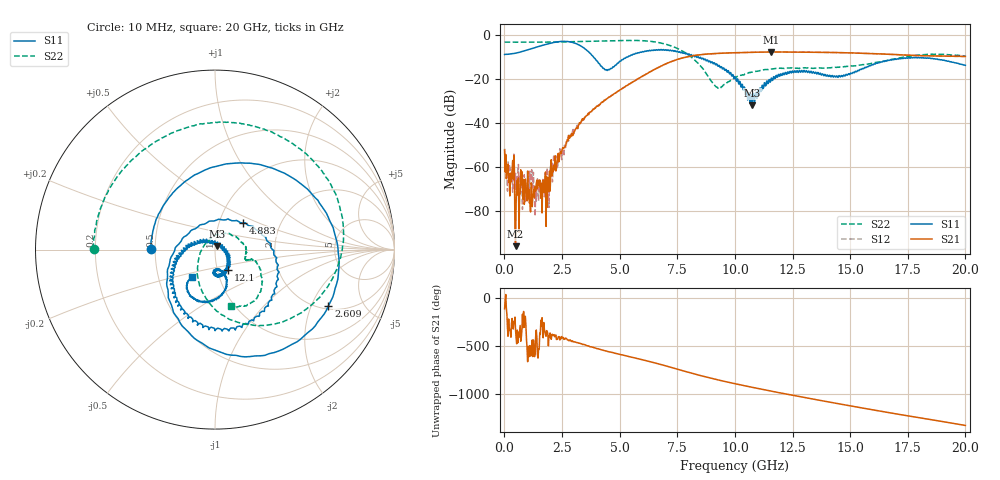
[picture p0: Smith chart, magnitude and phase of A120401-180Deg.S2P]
!  2-Port S-parameters saved by WinCal
! VAR MeasName=S-Parameters (CALIBRATED_DATA) read from VNA (N5244A)
! VAR MeasDate=11/21/2012 9:58:23 AM
! VAR NAME=A120401-180Deg
! VAR FILENAME=A120401-180Deg.S2P
! VAR DATE=11/21/2012 9:58:23 AM
! VAR PHYS_PORTS=1,2
# Hz S MA R 50
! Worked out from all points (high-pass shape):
!   801 points, 10 MHz to 20 GHz, reference 50 ohm
!   highest |S21| = -7.83 dB at 11.55 GHz (marker M1); lowest = -96.2 dB at 484.8 MHz (marker M2)
!   |S21| within 3 dB of the highest: 7.632 GHz to end of sweep
!   lowest |S11| = -32.1 dB at 10.75 GHz (marker M3), VSWR 1.05, Z = 51.3 + j2.13 ohm
!   |S11| at or under -10 dB: 3.858 GHz to 5.368 GHz (1.51 GHz wide, 32.7 % of centre); 8.329 GHz to 8.405 GHz (76.47 MHz wide, 0.914 % of centre); 8.406 GHz to end of sweep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
!   |S22| runs from -24.5 to -2.6 dB; largest |S21 - S12| = 0.0043
!   S11 on the Smith chart (normalised r, x): 10 MHz: 0.48, +0.00; 2.609 GHz: 2.14, -2.68; 4.883 GHz: 1.30, +0.41; 12.1 GHz: 1.13, -0.26; 20 GHz: 0.74, -0.24
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1e7  0.3546 179.4  0.002379 -112.7  0.002555 -35.3  0.6748 179.6
4.847625e8  0.3793 137.5  1.544e-05 26.9  0.0007012 -44.5  0.6757 168.2
8.59575e8  0.4268 107.0  0.0001381 54.4  0.0006519 97.2  0.6777 159.2
1.2094e9  0.4862 80.3  0.0001225 -77.3  0.000536 144.1  0.6797 150.8
1.384312e9  0.5201 67.7  0.0004048 25.9  0.0001636 141.6  0.6791 146.6
1.90905e9  0.6235 29.3  0.0005593 -137.9  0.0003853 57.3  0.6806 133.9
2.6087e9  0.7054 -26.5  0.002708 -62.7  0.003071 -51.4  0.6872 116.5
3.358325e9  0.5379 -95.5  0.01094 -118.3  0.01112 -121.8  0.7027 97.9
3.933038e9  0.2867 -157.3  0.02173 -160.1  0.02114 -160.9  0.7136 82.4
4.882562e9  0.2168 43.2  0.0497 140.5  0.04951 139.4  0.7323 53.8
6.681662e9  0.4568 -71.0  0.1808 33.7  0.1806 34.3  0.6647 -16.9
7.456275e9  0.4105 -105.6  0.2677 -18.2  0.2677 -18.3  0.5005 -57.6
8.330838e9  0.3152 -137.1  0.3411 -76.8  0.3408 -76.9  0.2434 -107.4
9.255375e9  0.1936 -169.1  0.3761 -132.4  0.3765 -132.2  0.06123 147.7
1.0005e10  0.1105 153.3  0.3887 -172.9  0.3906 -172.7  0.1059 59.1
1.075462e10  0.0248 56.6  0.3987 149.3  0.3981 149.5  0.141 26.4
1.155422e10  0.08789 -40.4  0.406 110.7  0.4057 110.7  0.1649 7.3
1.210395e10  0.1336 -56.2  0.4048 84.8  0.4053 84.7  0.1727 2.0
1.335332e10  0.1332 -89.6  0.4001 28.6  0.4004 28.4  0.1721 -9.0
1.525238e10  0.1462 -68.1  0.3829 -54.3  0.3832 -54.3  0.1971 -16.8
1.667666e10  0.2599 -83.2  0.3579 -114.1  0.3591 -114.2  0.267 -21.8
2e10  0.2011 -129.7  0.3203 112.2  0.3196 112.1  0.3273 -73.8
